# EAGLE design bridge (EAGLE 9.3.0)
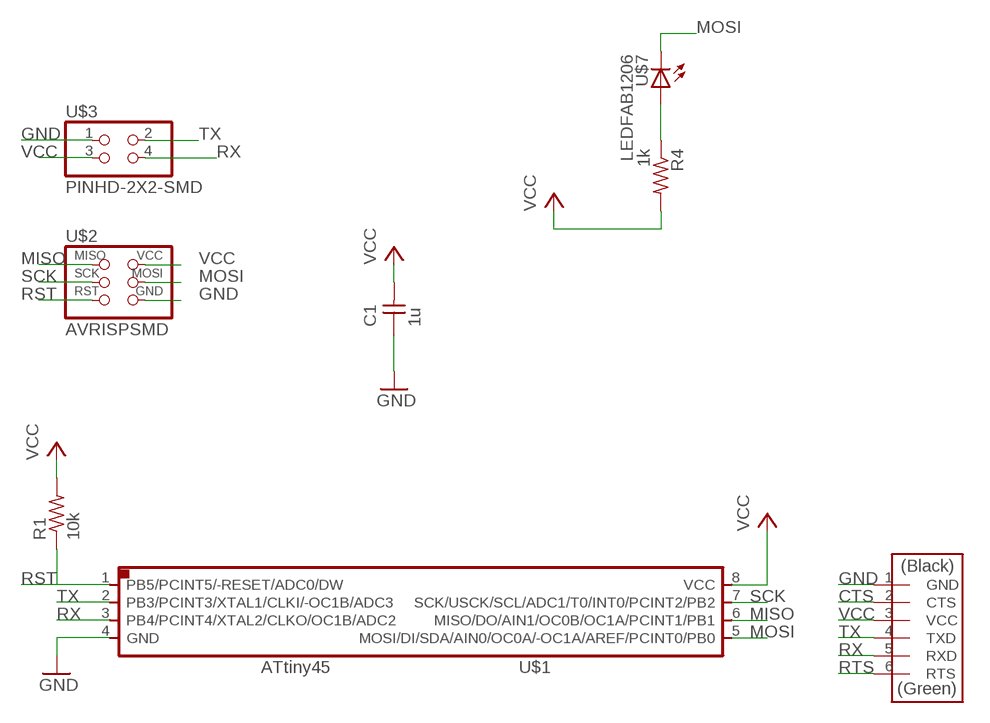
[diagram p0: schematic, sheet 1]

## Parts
C1  1u  CAP-UNPOLARIZEDFAB  [C1206FAB]
R1  10k  RES-US1206FAB  [R1206FAB]
R4  1k  RES-US1206FAB  [R1206FAB]
U$1  ATTINY45SI  [SOIC8]
U$2  AVRISPSMD  [2X03SMD]
U$3  PINHD-2X2-SMD  [2X02SMD]
U$4  FTDI-SMD-HEADER  [1X06SMD]
U$7  LEDFAB1206  [LED1206FAB]

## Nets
CTS: U$4.2(CTS)
GND: C1.1 U$1.4(GND) U$2.6(GND) U$3.1 U$4.1(GND)
MISO: U$1.6(MISO/DO/AIN1/OC0B/OC1A/PCINT1/PB1) U$2.1(MISO)
MOSI: U$1.5(MOSI/DI/SDA/AIN0/OC0A/-OC1A/AREF/PCINT0/PB0) U$2.4(MOSI) U$7.2(C)
N$4: R4.1 U$7.1(A)
RST: R1.1 U$1.1(PB5/PCINT5/-RESET/ADC0/DW) U$2.5(RST)
RTS: U$4.6(RTS)
RX: U$1.3(PB4/PCINT4/XTAL2/CLKO/OC1B/ADC2) U$3.4 U$4.5(RXD)
SCK: U$1.7(SCK/USCK/SCL/ADC1/T0/INT0/PCINT2/PB2) U$2.3(SCK)
TX: U$1.2(PB3/PCINT3/XTAL1/CLKI/-OC1B/ADC3) U$3.2 U$4.4(TXD)
VCC: C1.2 R1.2 R4.2 U$1.8(VCC) U$2.2(VCC) U$3.3 U$4.3(VCC)

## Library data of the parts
C1 = fab:CAP-UNPOLARIZED
R1 R4 = fab:RES-US: Resistor (US Symbol)
U$1 = fab:ATTINY45
U$2 = fab:AVRISP
U$3 = fab:PINHD-2X2-SMD
U$4 = fab:FTDI-SMD-HEADER
U$7 = fab:LED: LED

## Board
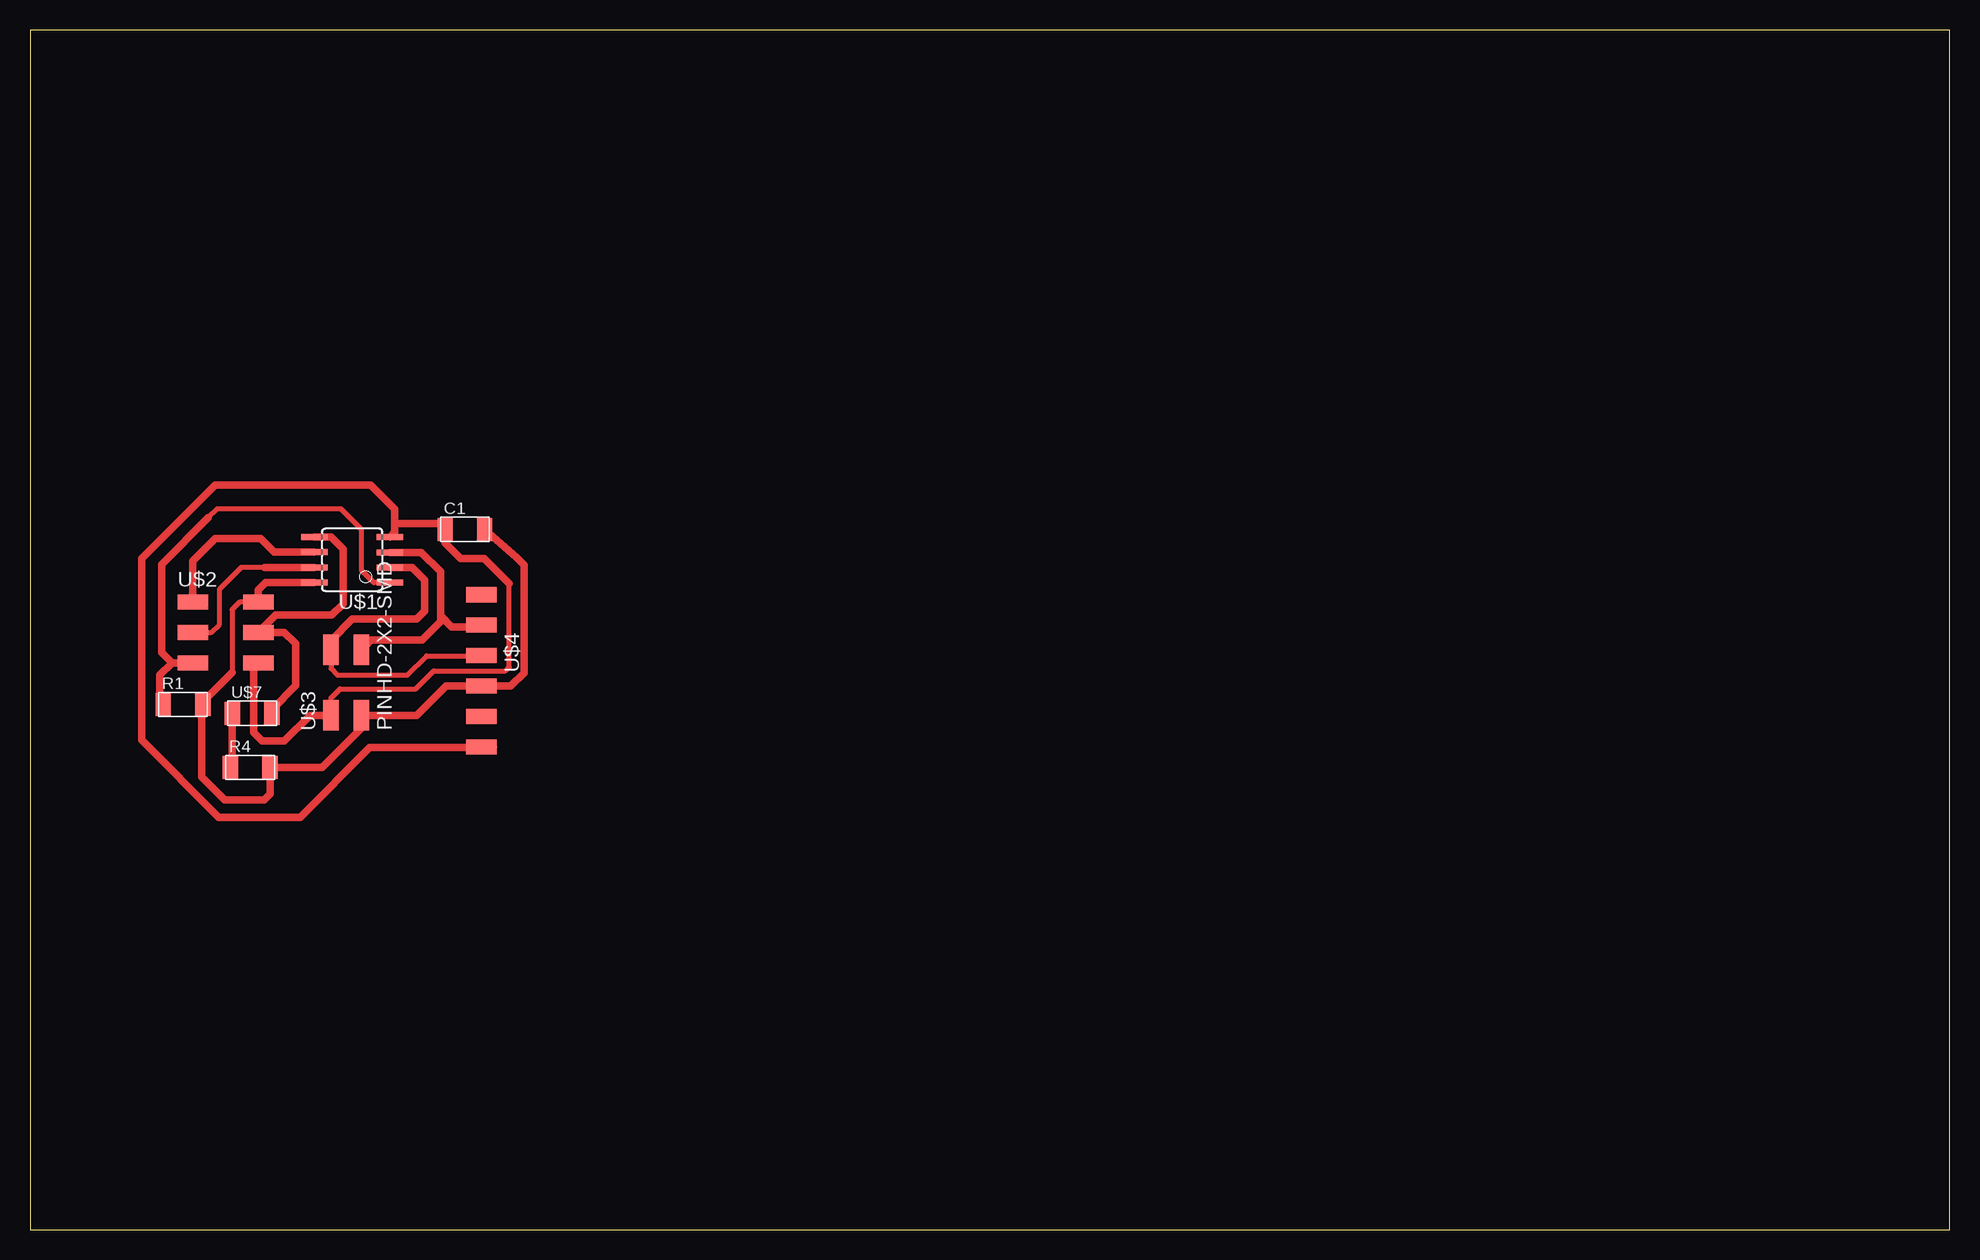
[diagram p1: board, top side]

Size 160 x 100 mm. Coordinates in mm from the lower left corner, seen from the top.
Outline: 0,0 160,0 160,100 0,100 0,0
Copper layers (1*16): Top 0.035mm / dielectric 1.5mm / Bottom 0.035mm
Design rules "default": minimum track width 6mil, minimum drill 0.35mm, track to track 6mil, track to pad 6mil, pad to pad 6mil, via to via 6mil, smd to smd 6mil, copper to edge 40mil, drill to drill 6mil, minimum pad ring 10mil, minimum via ring 8mil, stop-mask expansion 4mil, vias tented up to drill 0mil, thermal gap 10mil

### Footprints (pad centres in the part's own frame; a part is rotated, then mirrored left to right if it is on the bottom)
C1206FAB = smd 1.27 x 1.905: 1 -1.651,0; 2 1.651,0
R1206FAB = smd 1.27 x 1.905: 1 -1.651,0; 2 1.651,0
SOIC8 = smd 0.5 x 2.2: 1 -1.905,-3.154; 2 -0.645,-3.154; 3 0.625,-3.154; 4 1.895,-3.154; 5 1.905,3.154; 6 0.635,3.154; 7 -0.635,3.154; 8 -1.905,3.154
2X03SMD = smd 2.54 x 1.27: 1 -2.54,2.54; 2 2.92,2.54; 3 -2.54,0; 4 2.92,0; 5 -2.54,-2.54; 6 2.92,-2.54
2X02SMD = smd 2.54 x 1.27: 1 -2.54,1.27; 2 2.92,1.27; 3 -2.54,-1.27; 4 2.92,-1.27
1X06SMD = smd 2.54 x 1.27: 1 0,6.35; 2 0,3.81; 3 0,1.27; 4 0,-1.27; 5 0,-3.81; 6 0,-6.35
LED1206FAB = smd 1.27 x 1.905: 1 -1.651,0; 2 1.651,0

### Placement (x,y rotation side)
C1  36.25,58.36 0 top
R1  12.76,43.77 0 top
R4  18.35,38.52 0 top
U$1  26.86,55.83 90 top
U$2  16.12,49.77 0 top
U$3  26.35,45.41 90 top
U$4  37.61,46.58 180 top
U$7  18.52,43.03 0 top

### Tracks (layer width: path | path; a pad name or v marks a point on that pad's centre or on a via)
GND
  Top 0.406: 25.49,42.47 U$3.1 25.08,44.32 25.85,45.08 32.16,45.08 33.65,46.57 39.64,46.57 39.95,46.88 39.95,53.85 39.93,53.86
  Top 0.61: 37.54,40.16 U$4.1 | U$4.1 38.63,40.23 | U$2.6 18.64,46.83 18.64,41.44 19.36,40.71 21.2,40.71 23.36,42.87 U$3.1 25,42.78 | U$4.1 37.58,40.2 28.33,40.2 22.5,34.37 15.73,34.37 9.3,40.79 9.3,55.92 15.45,62.06 28.4,62.06 30.41,60.05 30.41,58.86 | 39.93,53.86 37.87,55.92 35.91,55.92 34.6,57.24 C1.1 34.1,58.86 30.41,58.86 | 30.41,58.86 30.41,58.13 U$1.4
MISO
  Top 0.61: U$1.6 20.34,56.47 19.21,57.59 15.46,57.59 13.58,55.72 U$2.1
MOSI
  Top 0.61: U$1.5 25.09,57.74 26.1,56.73 26.1,52.16 25.16,51.22 20.49,51.22 U$2.4 19.75,49.78 19.76,49.78 21.2,49.78 22.15,48.84 22.15,45.35 20.17,43.37 U$7.2
N$4
  Top 0.61: U$7.1 16.87,38.69 R4.1
RST
  Top 0.406: U$1.1 28.65,53.93 27.63,54.95 27.63,58.37 25.92,60.07 15.59,60.07 14.86,59.34
  Top 0.61: U$2.5 11.84,47.23 | 11.84,47.23 10.96,48.11 10.96,55.44 14.86,59.34 | R1.1 10.82,44.06 10.82,46.22 11.84,47.23
RX
  Top 0.61: U$3.4 28.44,49.15 32.68,49.15 34.22,50.69 34.22,51.18 | U$4.5 37.42,50.19 37.34,50.26 37.79,50.26 | 37.79,50.26 38.23,50.26 | 30.37,56.46 U$1.3 32.61,56.46 34.22,54.85 34.22,51.18 | 34.22,51.18 35.16,50.24 37.76,50.24 37.79,50.26
SCK
  Top 0.406: U$2.3 15.12,49.77 15.8,50.45 15.8,53.38 17.62,55.2 20.05,55.2
  Top 0.61: U$1.7 20.05,55.2 19.57,55.2
TX
  Top 0.406: U$3.2 25.08,46.76 25.62,46.22 31.44,46.22 33.05,47.83 37.6,47.83 U$4.4
  Top 0.61: U$1.2 31.87,55.19 32.91,54.14 32.91,51.56 32.23,50.88 26.87,50.88 25.08,49.1 U$3.2 | U$4.4 37.55,47.91
VCC
  Top 0.406: U$2.2 17.48,52.31 16.85,51.68 16.85,46.42
  Top 0.61: 20.04,38.48 R4.2 | 16.85,46.42 14.41,43.98 R1.2 14.33,43.69 14.33,37.72 16.23,35.82 19.52,35.82 20,36.3 R4.2 | U$1.8 19.65,53.93 19.04,53.32 U$2.2 | 38.58,45.3 U$4.3 | U$4.3 40.08,45.3 41.17,46.4 41.17,55.39 40.55,56.01 C1.2 | 36.69,45.3 U$4.3 | U$4.3 34.67,45.3 32.24,42.87 U$3.3 27.62,41.78 24.36,38.52 R4.2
